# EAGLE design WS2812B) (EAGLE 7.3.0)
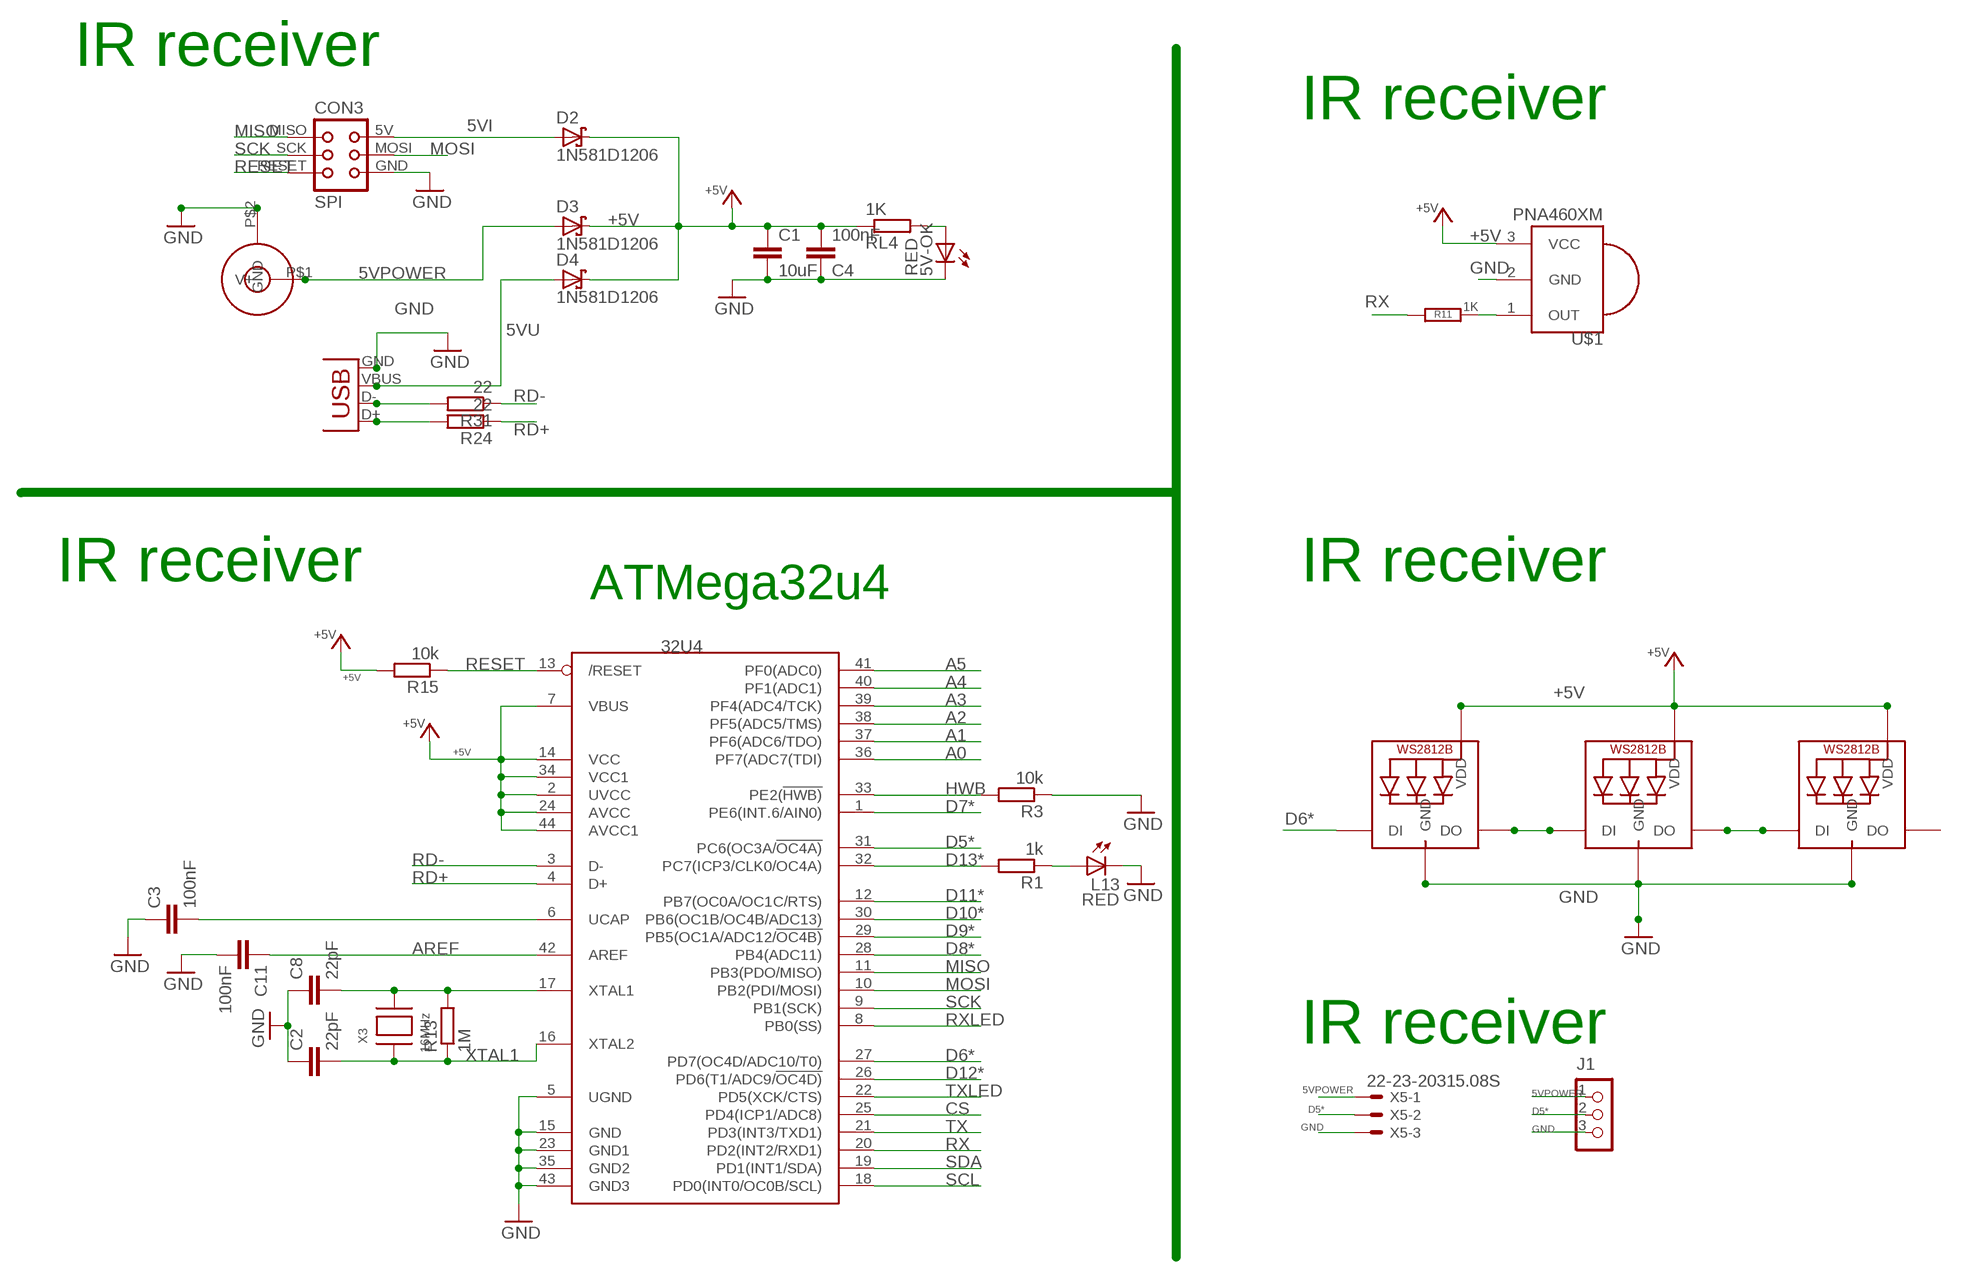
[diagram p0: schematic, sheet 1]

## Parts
5V-OK  RED  LEDCHIP-LED0805  [CHIP-LED0805]
C1  10uF  C-EUC1206  [C1206]
C2  22pF  C-EUC0805K  [C0805K]
C3  100nF  C-EUC0805K  [C0805K]
C4  100nF  C-EUC1206  [C1206]
C8  22pF  C-EUC0805K  [C0805K]
C11  100nF  C-EUC0805K  [C0805K]
CON2  JACK_DC_BARREL  [DC_BARREL]
CON3  SPI  TINYISPT  [TC2030-MCP-NL]
D2  1N581D1206  [LED-1206]
D3  1N581D1206  [LED-1206]
D4  1N581D1206  [LED-1206]
J1  CON_TERMINAL_BLOCK_03-5MM  [TERMINAL_BLOCK_3P_5]
L13  RED  LEDCHIP-LED0805  [CHIP-LED0805]
LED1  WS2812B_5050N  [WS2812B-NARROW]
LED2  WS2812B_5050N  [WS2812B-NARROW]
LED3  WS2812B_5050N  [WS2812B-NARROW]
R1  1k  R-EU_M0805  [M0805]
R3  10k  R-EU_M0805  [M0805]
R11  1K  R-EU_R0805  [R0805]
R13  1M  R-EU_M0805  [M0805]
R15  10k  R-EU_M0805  [M0805]
R24  22  R-EU_M0805  [M0805]
R31  22  R-EU_M0805  [M0805]
RL4  1K  R-EU_R0805  [R0805]
U$1  PNA460XM  [PNA460XM]
U$4  32U4  ATMEGA32U4-AU  [TQFP44]
X2  USB-MICROB  [USB-MICROB]
X3  16MHz  XTALNX6035  [NX6035]
X5  22-23-20315.08S  [3-PIN-5.08S]

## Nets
5VI: CON3.5V(VCC) D2.A
5VPOWER: CON2.P$1(V+) D3.A J1.1 X5.1
5VU: D4.A X2.VBUS
+5V [fine]: C1.1 C4.2 D2.C D3.C D4.C LED1.1-VDD(VDD) LED2.1-VDD(VDD) LED3.1-VDD(VDD) R15.2 RL4.1 U$1.3(VCC) U$4.2(UVCC) U$4.7(VBUS) U$4.14(VCC) U$4.24(AVCC) U$4.34(VCC1) U$4.44(AVCC1)
A0: U$4.36(PF7(ADC7(TDI))
A1: U$4.37(PF6(ADC6/TDO))
A2: U$4.38(PF5(ADC5/TMS))
A3: U$4.39(PF4(ADC4/TCK))
A4: U$4.40(PF1(ADC1))
A5: U$4.41(PF0(ADC0))
AREF: C11.1 U$4.42(AREF)
CS: U$4.25(PD4(ICP1/ADC8))
D5*: J1.2 U$4.31(PC6(OC3A/!OC4A)) X5.2
D6*: LED1.4-DIN(DI) U$4.27(PD7(OC4D/ADC10/T0))
D7*: U$4.1(PE6(INT.6/AIN0))
D8*: U$4.28(PB4(ADC11))
D9*: U$4.29(PB5(OC1A/ADC12/!OC4B))
D10*: U$4.30(PB6(OC1B/OC4B/ADC13))
D11*: U$4.12(PB7(OC0A/OC1C/RTS))
D12*: U$4.26(PD6(T1/ADC9/!OC4D))
D13*: R1.2 U$4.32(PC7(ICP3/CLK0/OC4A))
D_USB+ [USBA]: R24.2 X2.D+
D_USB- [USBA]: R31.2 X2.D-
GND [power]: 5V-OK.C C1.2 C2.1 C3.1 C4.1 C8.1 C11.2 CON2.P$2(GND) CON3.GND J1.3 L13.C LED1.3-GND(GND) LED2.3-GND(GND) LED3.3-GND(GND) R3.1 U$1.2(GND) U$4.5(UGND) U$4.15(GND) U$4.23(GND1) U$4.35(GND2) U$4.43(GND3) X2.GND X5.3
HWB: R3.2 U$4.33(PE2(!HWB))
MISO: CON3.MISO U$4.11(PB3(PDO/MISO))
MOSI: CON3.MOSI U$4.10(PB2(PDI/MOSI))
N$1: LED1.2-DOUT(DO) LED2.4-DIN(DI)
N$2: LED2.2-DOUT(DO) LED3.4-DIN(DI)
N$4: L13.A R1.1
N$9: R11.1 U$1.1(OUT)
N$12: 5V-OK.A RL4.2
N$16: C3.2 U$4.6(UCAP)
N$42: C8.2 R13.2 U$4.17(XTAL1) X3.P$2
RD+ [USBB]: R24.1 U$4.4(D+)
RD- [USBB]: R31.1 U$4.3(D-)
RESET: CON3.RESET R15.1 U$4.13(/RESET)
RX: R11.2 U$4.20(PD2(INT2/RXD1))
RXLED: U$4.8(PB0(SS))
SCK: CON3.SCK U$4.9(PB1(SCK))
SCL: U$4.18(PD0(INT0/OC0B/SCL))
SDA: U$4.19(PD1(INT1/SDA))
TX: U$4.21(PD3(INT3/TXD1))
TXLED: U$4.22(PD5(XCK/CTS))
XTAL1: C2.2 R13.1 U$4.16(XTAL2) X3.P$1
Unconnected: LED3.2-DOUT(DO)

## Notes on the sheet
- IR receiver
- IR receiver
- IR receiver | IR receiver
- ATMega32u4
- IR receiver

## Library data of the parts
5V-OK L13 = adafruit:LED: LED
C1-C4 C8 C11 = rcl:C-EU: CAPACITOR, European symbol
CON2 = lpatiny:JACK_DC_BARREL
CON3 = lpatiny:TINYISP: CONNECTOR
D2-D4 = lpatiny:1N581*: 1.0A SCHOTTKY BARRIER RECTIFIER
J1 = dp_devices:CON_TERMINAL_BLOCK_03: 3 poles, wire to board connector
LED1-LED3 = adafruit:WS2812B
R1 R3 R11 R15 RL4 = resistor:R-EU_: RESISTOR, European symbol
R13 R24 R31 = rcl:R-EU_: RESISTOR, European symbol
U$1 = adafruit:PNA460XM: IR 38KHz receiver PNA4602 and related receivers http://www.ladyada.net/library/pcb/eaglelibrary.html
U$4 = adafruit:ATMEGA32U4: http://www.ladyada.net/library/eagle
X2 = SparkFun:USB: USB Connectors USB-B-PTH is fully proven SKU : PRT-00139 USB-miniB is fully proven SKU : PRT-00587 USB-A-PCB is untested. USB-A-H is throughly reviewed, but untested. Spark Fun Electronics SKU : PRT-00437 USB-B-SMT is throughly reviewed, but untested. Needs silkscreen touching up. USB-A-S has not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
X3 = lpatiny:XTAL: Low cost SMT crystals, no capacitors included
X5 = lpatiny:22-23-2031: .100" (2.54mm) Center Header - 3 Pin

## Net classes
0 default: width 0.254 mm
1 power: width 0.254 mm
2 VIN: width 0.254 mm
3 fine: width 0.254 mm
4 aref: width 0.254 mm
5 USBA: width 0.254 mm, clearance 0.254 mm
6 USBB: width 0.254 mm, clearance 0.254 mm

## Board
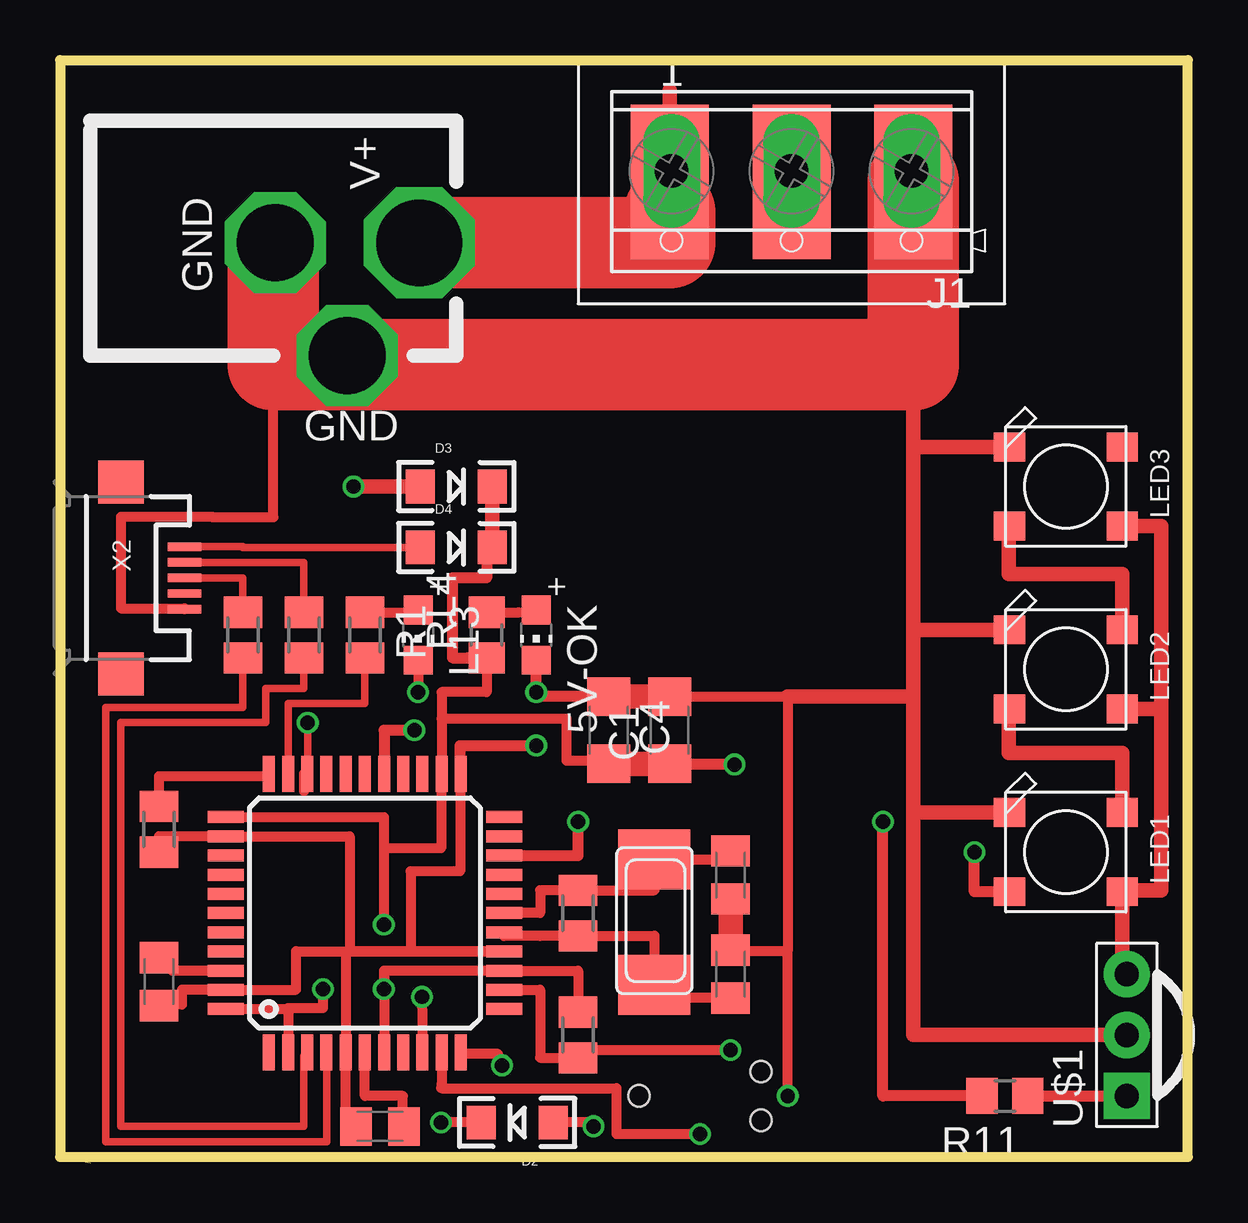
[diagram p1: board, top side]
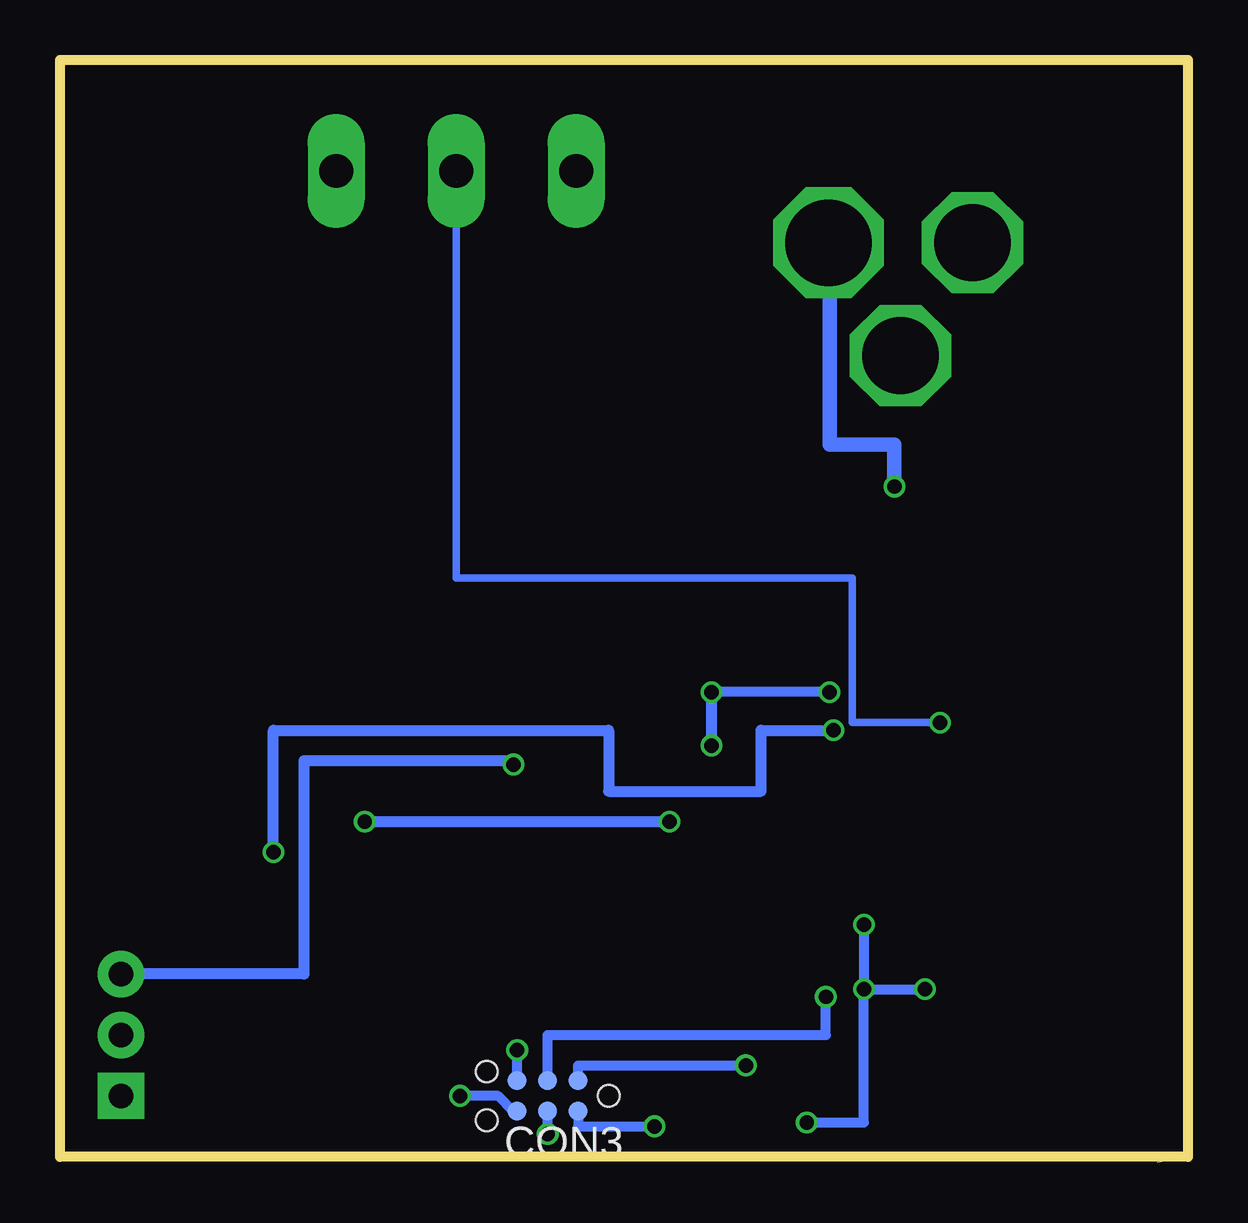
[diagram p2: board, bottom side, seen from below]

Size 46.99 x 45.97 mm. Coordinates in mm from the lower left corner, seen from the top.
Outline: 0,0.25 1.27,0
Outline: 0,0.25 46.99,0.25 46.99,45.97 0,45.97 0,0.25
Copper layers (1*16): Top 0.035mm / dielectric 1.5mm / Bottom 0.035mm
Design rules "Fusion_eagle_rule_v1.1": minimum track width 6mil, minimum drill 12mil, track to track 6mil, track to pad 6mil, pad to pad 6mil, via to via 6mil, smd to smd 0mil, copper to edge 10mil, drill to drill 10mil, minimum pad ring 10mil, minimum via ring 6mil, stop-mask expansion 2mil, vias tented up to drill 100mil, thermal gap 10mil
vRestrict: area 5.1,2.8 to 20.3,6.6; area 5.1,2.8 to 8.9,16.8; area 16.5,5.3 to 20.3,18; area 5.1,14.2 to 20.3,18; area 22.9,0.9 to 30.5,4.7

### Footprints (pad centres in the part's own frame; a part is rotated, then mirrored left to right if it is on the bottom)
CHIP-LED0805 = smd 1.2 x 1.2: A 0,-1.05; C 0,1.05
C1206 = smd 1.6 x 1.8: 1 -1.4,0; 2 1.4,0
C0805K = smd 1.3 x 1.6: 1 -1,0; 2 1,0
DC_BARREL = drill 3.6 pad 4.5 octagon: P$1 0,13.7 | drill 3.2 pad 4.064 octagon: P$2 0,7.7; P$3 4.7,10.7
TC2030-MCP-NL = smd 0.787 x 0.787: 5V 1.27,0.635; GND 3.81,0.635; MISO 1.27,-0.635; MOSI 2.54,0.635; RESET 3.81,-0.635; SCK 2.54,-0.635 | hole 0.889: 0,0; 5.08,-1.016; 5.08,1.016
LED-1206 = smd 1.2 x 1.4: A -1.5,0; C 1.5,0
TERMINAL_BLOCK_3P_5 = drill 1.4 pad 2.38 long: 1 5,-0.45; 2 0,-0.45; 3 -5,-0.45
WS2812B-NARROW = smd 1.3 x 1.2: 1-VDD 2.35,-1.65; 2-DOUT 2.35,1.65; 3-GND -2.35,1.65; 4-DIN -2.35,-1.65
M0805 = smd 1.3 x 1.6: 1 -0.95,0; 2 0.95,0
R0805 = smd 1.3 x 1.5: 1 -0.95,0; 2 0.95,0
PNA460XM = drill 1.016 pad 1.93 square: 1 -2.54,0 | drill 1.016 pad 1.93: 2 0,0; 3 2.54,0
TQFP44 = smd 1.5 x 0.5: 1 -5.8,4; 2 -5.8,3.2; 3 -5.8,2.4; 4 -5.8,1.6; 5 -5.8,0.8; 6 -5.8,0; 7 -5.8,-0.8; 8 -5.8,-1.6; 9 -5.8,-2.4; 10 -5.8,-3.2; 11 -5.8,-4; 23 5.8,-4; 24 5.8,-3.2; 25 5.8,-2.4; 26 5.8,-1.6; 27 5.8,-0.8; 28 5.8,0; 29 5.8,0.8; 30 5.8,1.6; 31 5.8,2.4; 32 5.8,3.2; 33 5.8,4 | smd 0.5 x 1.5: 12 -4,-5.8; 13 -3.2,-5.8; 14 -2.4,-5.8; 15 -1.6,-5.8; 16 -0.8,-5.8; 17 0,-5.8; 18 0.8,-5.8; 19 1.6,-5.8; 20 2.4,-5.8; 21 3.2,-5.8; 22 4,-5.8; 34 4,5.8; 35 3.2,5.8; 36 2.4,5.8; 37 1.6,5.8; 38 0.8,5.8; 39 0,5.8; 40 -0.8,5.8; 41 -1.6,5.8; 42 -2.4,5.8; 43 -3.2,5.8; 44 -4,5.8
USB-MICROB = smd 0.35 x 1.4: D+ 0,2.65; D- -0.65,2.65; GND 1.3,2.65; ID 0.65,2.65; VBUS -1.3,2.65 | smd 1.8 x 1.9: MT1 -4,0; MT2 4,0
NX6035 = smd 2.5 x 3: P$1 2.665,0; P$2 -2.565,0
3-PIN-5.08S = smd 3.251 x 6.452: 1 -5.08,0; 2 0,0; 3 5.08,0

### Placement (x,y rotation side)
5V-OK  19.84,22 180 top
C1  25.4,18.03 90 top
C2  27.94,7.87 270 top
C3  13.33,1.52 0 top
C4  22.86,18.03 270 top
C8  27.94,12 90 top
C11  4.13,7.56 270 top
CON2  1.27,38.35 270 top
CON3  24.13,2.79 180 bottom
D2  19.05,1.68 180 top
D3  16.51,28.19 0 top
D4  16.51,25.65 0 top
J1  30.48,40.89 180 top
L13  14.92,22 180 top
LED1  41.91,12.95 0 top
LED2  41.91,20.57 0 top
LED3  41.91,28.19 0 top
R1  12.7,22 270 top
R3  4.13,13.91 90 top
R11  39.37,2.79 180 top
R13  21.59,10.41 90 top
R15  21.59,5.33 90 top
R24  7.62,22 90 top
R31  10.16,22 90 top
RL4  17.78,22 90 top
U$1  44.45,5.33 90 top
U$4  12.7,10.41 90 top
X2  2.54,24.38 270 top
X3  24.77,10.1 270 top
X5  30.48,40.89 0 top

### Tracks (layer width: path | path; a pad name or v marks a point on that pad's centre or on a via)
5VI  (via drill 0.6)
  Top 0.406: v22.22,1.52 22.07,1.68 D2.A
  Bottom 0.406: CON3.5V 25.4,1.52 v22.22,1.52
5VPOWER  (via drill 0.6)
  Top 0.305: 25.4,41.34 X5.1
  Top 0.457: X5.1 25.4,38.35
  Top 0.61: J1.1 25.4,41.34 25.4,44.7 | v12.22,28.19 D3.A
  Top 3.81: CON2.P$1 25.4,38.35 25.4,39.62
  Bottom 0.61: CON2.P$1 14.92,38.35 14.92,29.94 12.22,29.94 v12.22,28.19
5VU
  Top 0.305: X2.VBUS 7.62,25.68 7.62,25.65 D4.A
+5V  (via drill 0.6)
  Top 0.406: U$4.44 9.5,6.41 | 9.5,6.41 U$4.2 | U$4.14 13.5,8.01 U$4.7 | U$4.14 13.49,8.01 v13.49,7.24 | v10.95,7.24 10.95,6.45 9.5,6.45 9.5,6.41 | 13.49,13.11 15.88,13.11 15.88,16.21 U$4.24 15.9,18.51 | 13.49,13.11 v13.49,9.94 | U$4.34 13.49,14.41 13.49,13.11 | U$4.14 21.59,8.01 R15.2 | D2.C v15.88,1.68 | RL4.1 17.78,19.62 15.9,19.62 15.9,18.51 | 22.86,16.76 21.11,16.76 21.11,18.51 15.9,18.51
  Top 0.457: D4.C 17.78,25.65 17.78,24.38 16.35,24.38 16.35,21.05 16.99,21.05 RL4.1 | C1.1 28.1,16.63 v28.1,16.61
  Top 0.61: D3.C D4.C | C4.2 22.86,16.76 | LED2.1-VDD 45.88,18.92 | 45.88,18.92 45.88,11.37 44.26,11.37 LED1.1-VDD 44.26,7.87 U$1.3 | LED3.1-VDD 45.88,26.54 45.88,18.92
  Top 1.016: C1.1 C4.2
  Bottom 0.406: v13.49,7.24 v10.95,7.24 | v13.49,9.94 v13.49,7.24 | v15.88,1.68 13.49,1.68 v13.49,7.24
  Bottom 0.457: v28.1,16.61 27.94,16.61 27.94,16.76 36.83,16.76 36.83,7.87 U$1.3
AREF
  Top 0.406: U$4.42 4.67,8.01 C11.1
D5*  (via drill 0.6)  (1 unrouted)
  Top 0.305: U$4.31 10.32,16.21 v10.32,18.35
  Top 0.406: U$4.31 10.16,16.21 10.16,15.49
  Top 0.457: J1.2 X5.2 30.48,38.35
  Bottom 0.305: v10.32,18.35 13.97,18.35 13.97,24.38 30.48,24.38 X5.2
D6*  (via drill 0.6)
  Top 0.457: LED1.4-DIN 38.1,11.3 v38.1,12.95 | v14.76,18.03 13.5,18.03 | 13.49,18.03 13.5,18.03 | 13.5,18.03 U$4.27
  Bottom 0.457: v38.1,12.95 38.1,18.03 24.13,18.03 24.13,15.49 17.78,15.49 17.78,18.03 v14.76,18.03
D13*
  Top 0.305: R1.2 12.7,19.14 9.5,19.14 U$4.32
D_USB+
  Top 0.305: R24.2 7.62,24.38 X2.D+
D_USB-
  Top 0.305: X2.D- 10.16,25.03 R31.2
GND  (via drill 0.6)
  Top 0.406: 27.94,9.14 C2.1 27.99,8.83 30.32,8.83 | X2.GND 5.19,23.11 2.54,23.11 2.54,26.92 6.35,26.92 8.89,26.92 8.89,34.54 | C3.1 11.9,1.52 U$4.5 11.9,8.81 U$4.15 18.5,8.83 14.61,8.83 | 12.06,8.83 9.84,8.83 9.84,7.21 U$4.43 5.08,7.21 5.08,6.6 4.13,6.6 C11.2 | 12.06,8.83 14.61,8.83 | 12.06,8.83 12.06,13.61 U$4.35 4.13,13.61 R3.1 | U$4.23 16.67,16.21 16.67,12.16 14.61,12.16 14.61,8.83 | v30.32,2.79 30.32,8.83 | L13.C v14.92,19.62 | v19.84,19.62 19.84,19.43 | C1.2 30.32,19.43 30.32,8.83
  Top 0.457: C4.1 19.84,19.43 5V-OK.C | J1.3 35.48,40.97 X5.3 35.56,29.46 | 16.67,16.21 16.67,17.4 v19.84,17.4
  Top 0.61: LED3.3-GND 35.56,29.84 | 35.56,29.84 35.56,33.27 | LED2.3-GND 35.56,22.22 | 35.56,22.22 35.56,29.46 35.56,29.84 | LED1.3-GND 35.56,14.6 | 35.56,14.6 35.56,19.43 | 35.56,19.43 35.56,22.22 | U$1.2 35.56,5.33 35.56,14.6 | 30.32,19.43 35.56,19.43
  Top 1.016: C1.2 C4.1 | C8.1 27.94,9.14
  Top 3.81: CON2.P$2 8.89,38.35 8.89,34.54 8.89,33.27 35.56,33.27 X5.3
  Bottom 0.406: CON3.GND 28.1,2.16 28.73,2.79 v30.32,2.79 | v14.92,19.62 v19.84,19.62
  Bottom 0.457: v19.84,17.4 v19.84,19.62
HWB
  Top 0.406: R3.2 4.13,16.13 8.7,16.13 U$4.33
MISO  (via drill 0.6)
  Top 0.406: v18.41,4.06 18.26,4.06 18.26,4.54 16.7,4.54 U$4.11
  Bottom 0.406: CON3.MISO 25.4,4.06 v18.41,4.06
MOSI  (via drill 0.6)
  Top 0.406: U$4.10 15.9,3.29 15.88,3.11 23.18,3.11 23.18,1.21 v26.67,1.21
  Bottom 0.406: v26.67,1.21 CON3.MOSI
N$1
  Top 0.61: LED2.4-DIN 39.53,18.92 39.53,17.08 44.26,17.08 LED1.2-DOUT
N$2
  Top 0.61: LED3.4-DIN 39.53,26.54 39.53,24.54 44.26,24.54 LED2.2-DOUT
N$4
  Top 0.406: R1.1 14.82,22.95 L13.A
N$9
  Top 0.457: R11.1 U$1.1
N$12
  Top 0.406: RL4.2 19.11,22.95 5V-OK.A
N$16
  Top 0.406: C3.2 14.29,1.52 14.29,2.79 12.7,2.79 U$4.6
N$42
  Top 0.406: U$4.17 20,10.41 20,11.36 R13.2 24.77,11.36 X3.P$2 27.94,12.66 C8.2
RD+
  Top 0.305: R24.1 7.62,18.99 1.91,18.99 1.91,0.89 11.11,0.89 11.11,4.6 U$4.4
RD-
  Top 0.305: U$4.3 10.16,4.47 10.16,1.52 2.54,1.52 2.54,18.35 8.57,18.35 8.57,19.78 10.16,19.78 R31.1
RESET  (via drill 0.6)
  Top 0.406: U$4.13 20,7.21 20,4.38 R15.1 21.59,4.7 v27.94,4.7
  Bottom 0.406: CON3.RESET v27.94,4.7
RX  (via drill 0.6)
  Top 0.457: R11.2 34.29,2.79 v34.29,14.22 | U$4.20 21.59,12.81 v21.59,14.22
  Bottom 0.457: v21.59,14.22 v34.29,14.22
SCK  (via drill 0.6)
  Top 0.406: v15.08,6.92 15.1,5.97 U$4.9
  Bottom 0.406: CON3.SCK 26.67,5.33 15.08,5.33 v15.08,6.92
XTAL1
  Top 0.406: U$4.16 18.5,9.46 20,9.46 R13.1 24.77,9.46 X3.P$1 24.77,6.87 C2.2

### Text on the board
tDocu: 5V | OUT | GND | Led control v1.0
203bmp: C:/Users/G/Pictures/logo_epfl.bmp

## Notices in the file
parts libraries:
lpatiny: ©2009 ROFA.cz - modified and updated by Robert Darlington ‹rdarlington@gmail.com›
SparkFun: Licensing: CC v3.0 Share-Alike You are welcome to use this library for commercial purposes.
